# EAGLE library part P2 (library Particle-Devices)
Particle P2 module (WiFi with antenna)
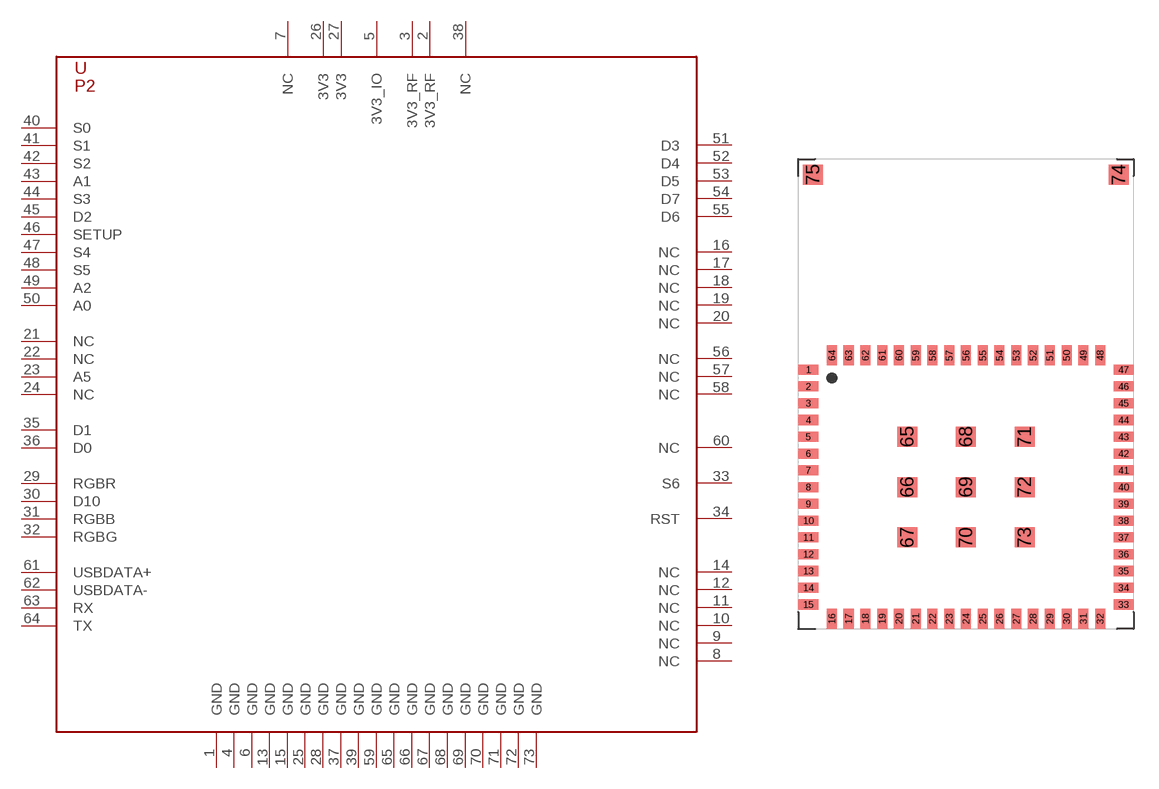
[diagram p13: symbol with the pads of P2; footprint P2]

Designator prefix U

## P2  [P2]
1  GND
2  3V3_RF
3  3V3_RF
4  GND
5  3V3_IO
6  GND
7  NC
8  NC
9  NC
10  NC
11  NC
12  NC
13  GND
14  NC
15  GND
16  NC
17  NC
18  NC
19  NC
20  NC
21  NC
22  NC
23  A5
24  NC
25  GND
26  3V3
27  3V3
28  GND
29  RGBR
30  D10
31  RGBB
32  RGBG
33  S6
34  RST
35  D1
36  D0
37  GND
38  NC
39  GND
40  S0
41  S1
42  S2
43  A1
44  S3
45  D2
46  SETUP
47  S4
48  S5
49  A2
50  A0
51  D3
52  D4
53  D5
54  D7
55  D6
56  NC
57  NC
58  NC
59  GND
60  NC
61  USBDATA+
62  USBDATA-
63  RX
64  TX
65  GND
66  GND
67  GND
68  GND
69  GND
70  GND
71  GND
72  GND
73  GND

## Footprint P2 (pad centres in mm)
smd 1.2 x 0.6: 1 0.6,15.45; 2 0.6,14.45; 3 0.6,13.45; 4 0.6,12.45; 5 0.6,11.45; 6 0.6,10.45; 7 0.6,9.45; 8 0.6,8.45; 9 0.6,7.45; 10 0.6,6.45; 11 0.6,5.45; 12 0.6,4.45; 13 0.6,3.45; 14 0.6,2.45; 15 0.6,1.45; 33 19.4,1.45; 34 19.4,2.45; 35 19.4,3.45; 36 19.4,4.45; 37 19.4,5.45; 38 19.4,6.45; 39 19.4,7.45; 40 19.4,8.45; 41 19.4,9.45; 42 19.4,10.45; 43 19.4,11.45; 44 19.4,12.45; 45 19.4,13.45; 46 19.4,14.45; 47 19.4,15.45
smd 0.6 x 1.2: 16 2,0.6; 17 3,0.6; 18 4,0.6; 19 5,0.6; 20 6,0.6; 21 7,0.6; 22 8,0.6; 23 9,0.6; 24 10,0.6; 25 11,0.6; 26 12,0.6; 27 13,0.6; 28 14,0.6; 29 15,0.6; 30 16,0.6; 31 17,0.6; 32 18,0.6; 48 18,16.3; 49 17,16.3; 50 16,16.3; 51 15,16.3; 52 14,16.3; 53 13,16.3; 54 12,16.3; 55 11,16.3; 56 10,16.3; 57 9,16.3; 58 8,16.3; 59 7,16.3; 60 6,16.3; 61 5,16.3; 62 4,16.3; 63 3,16.3; 64 2,16.3
smd 1.2 x 1.2: 65 6.5,11.45; 66 6.5,8.45; 67 6.5,5.45; 68 10,11.45; 69 10,8.45; 70 10,5.45; 71 13.5,11.45; 72 13.5,8.45; 73 13.5,5.45; 74 19.12,27.07; 75 0.88,27.07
